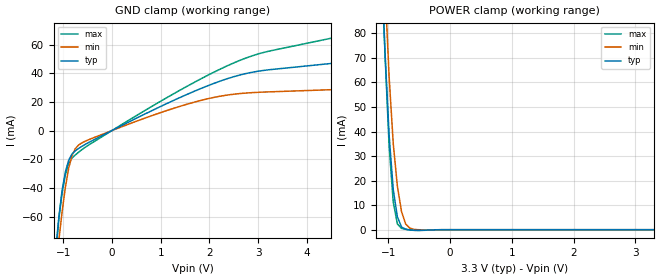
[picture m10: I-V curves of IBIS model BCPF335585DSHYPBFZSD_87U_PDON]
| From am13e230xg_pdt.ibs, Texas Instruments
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|   Model BCPF335585DSHYPBFZSD_87U_PDON
[Model] BCPF335585DSHYPBFZSD_87U_PDON
Model_type Input
Polarity   Non-Inverting
Enable   Active-High
Vinl =  0.990V
Vinh =  2.310V
C_comp   0.815pF   0.757pF   0.879pF
[Model Spec]
Vinh   2.310V   2.079V   2.541V
Vinl   0.990V   0.891V   1.089V
[Temperature Range]   25.000   0.155k   -40.000
[Voltage Range]   3.300V   2.970V   3.630V
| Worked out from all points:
|   GND clamp passes 1 mA (typ) near -0.06 V on its own axis
|   POWER clamp passes 1 mA (typ) near -0.78 V on its own axis
[GND_clamp]
|Voltage   I(typ)   I(min)   I(max)
-3.3V     -1.054A    -926mA     -1.327A
-1.156V   -83.43mA   -97.53mA   -87.3mA
-1.089V   -60.01mA   -75.98mA   -60.99mA
-1.022V   -41.21mA   -56.2mA    -43.04mA
-955mV    -28.58mA   -39.18mA   -30.66mA
-888mV    -20.7mA    -26.13mA   -22.63mA
-821mV    -16.36mA   -17.57mA   -19.18mA
-687mV    -12.53mA   -10.19mA   -15.17mA
1.39V     22.94mA    16.82mA    28.02mA
2.395V    36.46mA    24.87mA    45.59mA
3.132V    42.02mA    26.85mA    54.63mA
6.6V      53.99mA    30.98mA    79.2mA
[POWER_clamp]
|Voltage   I(typ)   I(min)   I(max)
-3.3V     1.803A     2.051A     1.936A
-1.122V   113.2mA    143.1mA    117.4mA
-1.055V   72.37mA    99.36mA    72.02mA
-988mV    38.58mA    62.43mA    34.24mA
-921mV    16.33mA    35.14mA    11.28mA
-854mV    5.234mA    17.71mA    2.369mA
-787mV    1.093mA    7.407mA    547.7uA
-720mV    204.9uA    2.351mA    147uA
-653mV    -56.63uA   652.4uA    -112.4uA
-519mV    -241.5uA   594.8nA    -325.8uA
-117mV    0A         0A         0A
3.3V      0A         0A         0A
